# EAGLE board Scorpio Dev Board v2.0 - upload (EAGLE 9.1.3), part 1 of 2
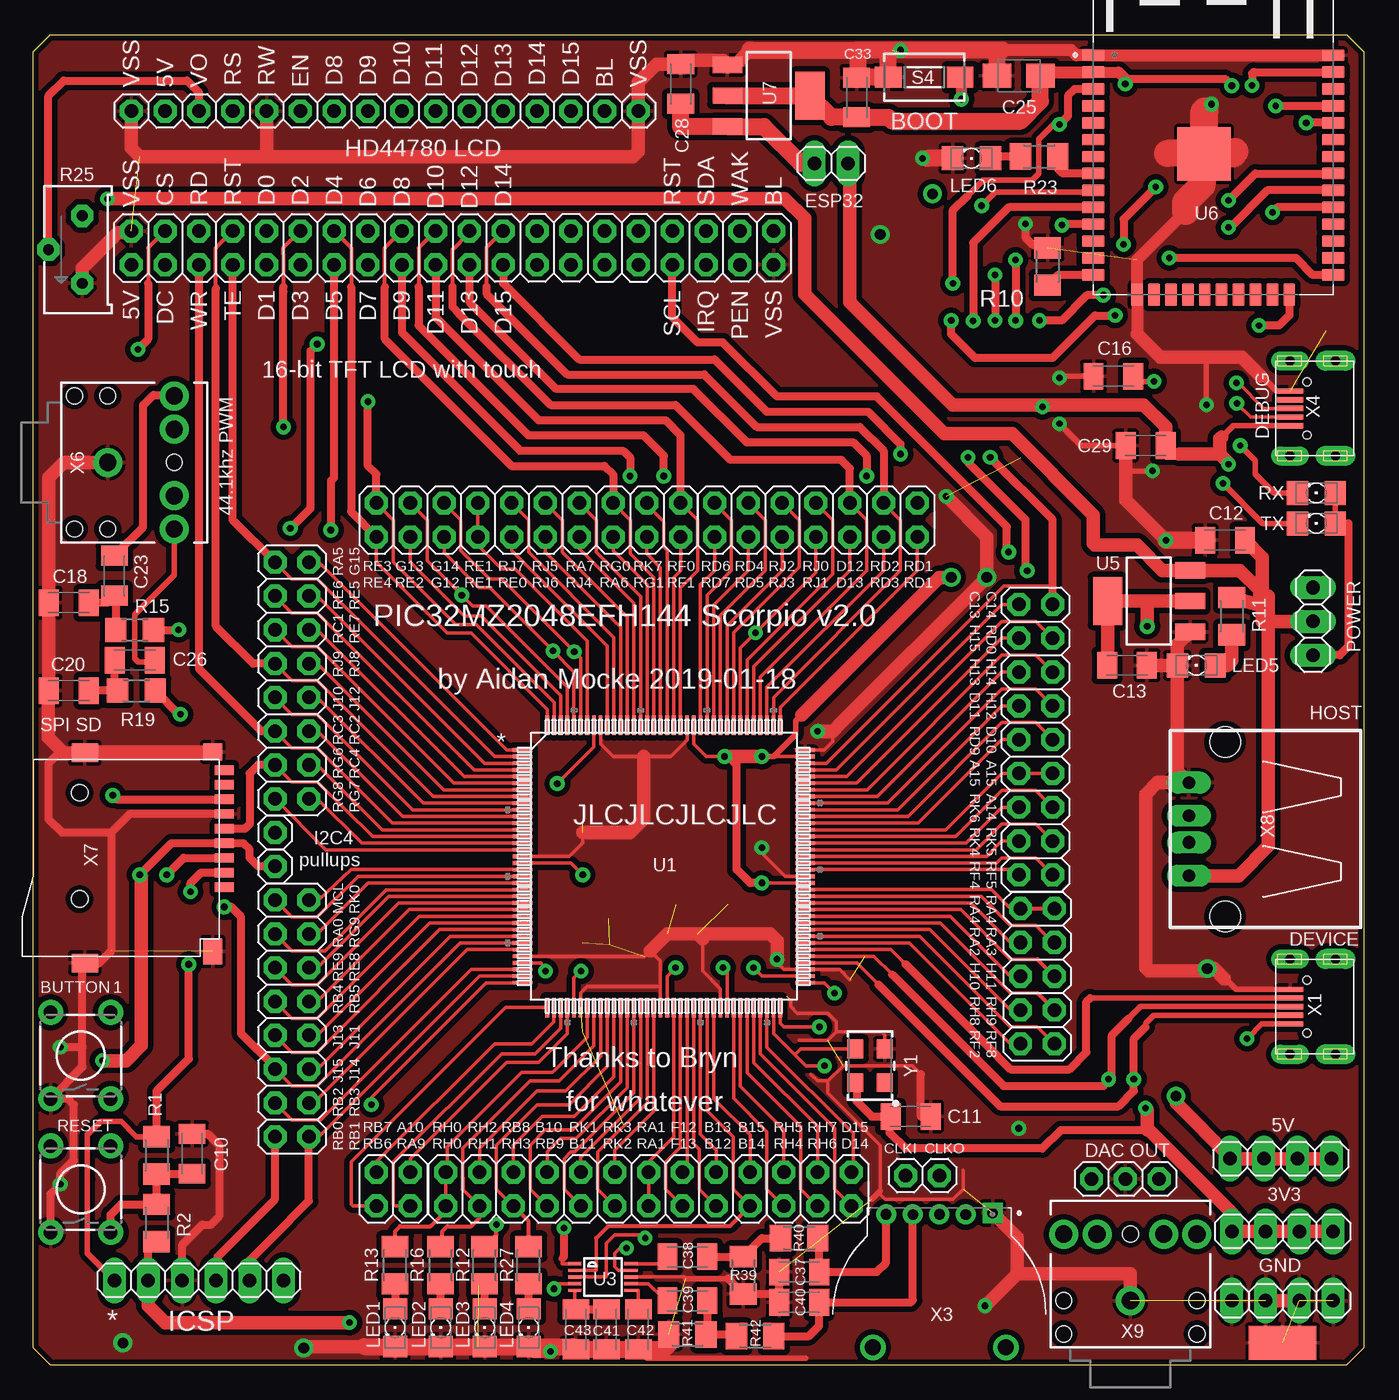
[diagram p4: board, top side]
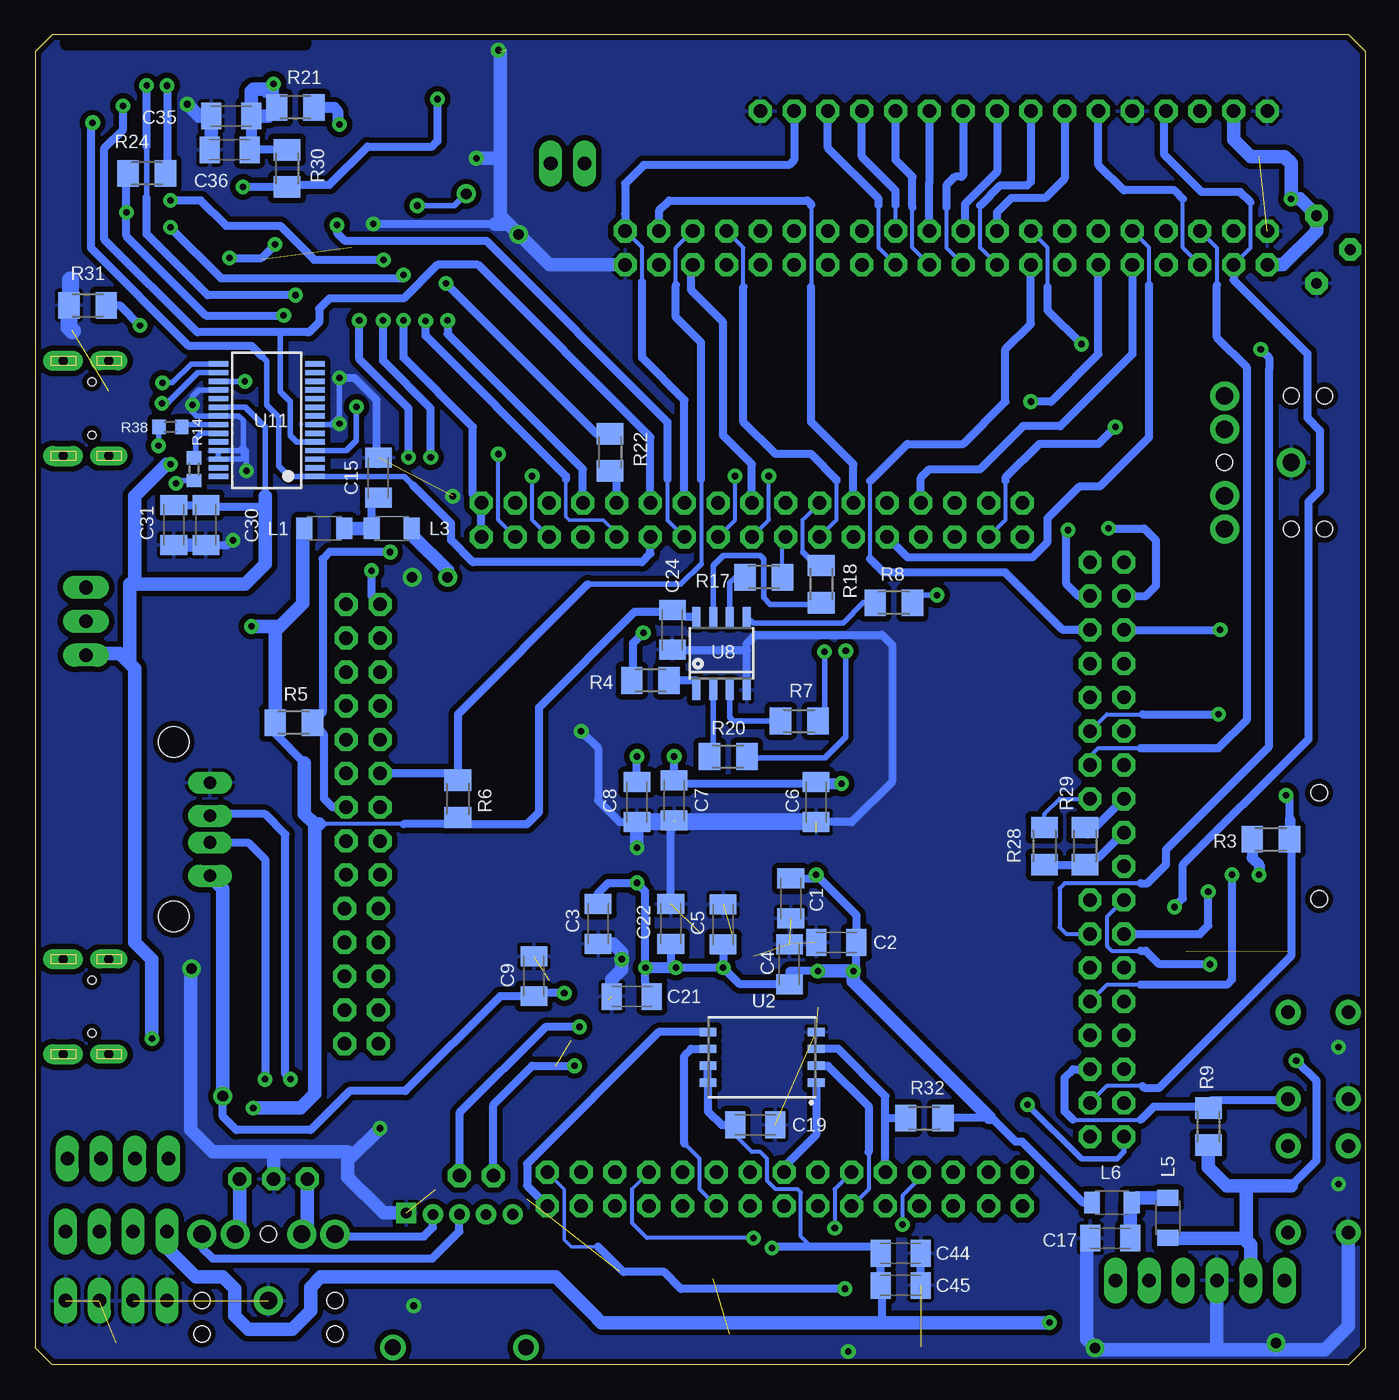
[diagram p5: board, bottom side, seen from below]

Size 99.95 x 99.95 mm. Coordinates in mm from the lower left corner, seen from the top.
Outline: 98.68,0 99.95,1.27 99.95,98.68 98.68,99.95 1.27,99.95 0,98.68 0,1.27 1.27,0 98.68,0
Copper layers (1*16): Top 0.035mm / dielectric 1.5mm / Bottom 0.035mm
Design rules "default *": minimum track width 10mil, minimum drill 19mil, track to track 7mil, track to pad 7mil, pad to pad 7mil, via to via 7mil, smd to smd 7mil, copper to edge 12mil, drill to drill 8mil, minimum pad ring 14mil, minimum via ring 12mil, stop-mask expansion 4mil, vias tented up to drill 0mil, thermal gap 10mil

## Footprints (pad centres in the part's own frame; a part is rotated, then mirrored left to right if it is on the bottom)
C1206K = smd 1.5 x 2: 1 -1.5,0; 2 1.5,0
B/3528-21W = smd 2.15 x 1.8: + 1.625,0; - -1.625,0
2X02 = drill 1.016 octagon: 1 -1.27,-1.27; 2 -1.27,1.27; 3 1.27,-1.27; 4 1.27,1.27
1X01 = drill 1.016 octagon: 1 0,0
2X07 = drill 1.016 octagon: 1 -7.62,-1.27; 2 -7.62,1.27; 3 -5.08,-1.27; 4 -5.08,1.27; 5 -2.54,-1.27; 6 -2.54,1.27; 7 0,-1.27; 8 0,1.27; 9 2.54,-1.27; 10 2.54,1.27; 11 5.08,-1.27; 12 5.08,1.27; 13 7.62,-1.27; 14 7.62,1.27
2X05 = drill 1.016 octagon: 1 -5.08,-1.27; 2 -5.08,1.27; 3 -2.54,-1.27; 4 -2.54,1.27; 5 0,-1.27; 6 0,1.27; 7 2.54,-1.27; 8 2.54,1.27; 9 5.08,-1.27; 10 5.08,1.27
2X20 = drill 1.016 octagon: 1 -24.13,-1.27; 2 -24.13,1.27; 3 -21.59,-1.27; 4 -21.59,1.27; 5 -19.05,-1.27; 6 -19.05,1.27; 7 -16.51,-1.27; 8 -16.51,1.27; 9 -13.97,-1.27; 10 -13.97,1.27; 11 -11.43,-1.27; 12 -11.43,1.27; 13 -8.89,-1.27; 14 -8.89,1.27; 15 -6.35,-1.27; 16 -6.35,1.27; 17 -3.81,-1.27; 18 -3.81,1.27; 19 -1.27,-1.27; 20 -1.27,1.27; 21 1.27,-1.27; 22 1.27,1.27; 23 3.81,-1.27; 24 3.81,1.27; 25 6.35,-1.27; 26 6.35,1.27; 27 8.89,-1.27; 28 8.89,1.27; 29 11.43,-1.27; 30 11.43,1.27; 31 13.97,-1.27; 32 13.97,1.27; 33 16.51,-1.27; 34 16.51,1.27; 35 19.05,-1.27; 36 19.05,1.27; 37 21.59,-1.27; 38 21.59,1.27; 39 24.13,-1.27; 40 24.13,1.27
2X08 = drill 1.016 octagon: 1 -8.89,-1.27; 2 -8.89,1.27; 3 -6.35,-1.27; 4 -6.35,1.27; 5 -3.81,-1.27; 6 -3.81,1.27; 7 -1.27,-1.27; 8 -1.27,1.27; 9 1.27,-1.27; 10 1.27,1.27; 11 3.81,-1.27; 12 3.81,1.27; 13 6.35,-1.27; 14 6.35,1.27; 15 8.89,-1.27; 16 8.89,1.27
2X03 = drill 1.016 octagon: 1 -2.54,-1.27; 2 -2.54,1.27; 3 0,-1.27; 4 0,1.27; 5 2.54,-1.27; 6 2.54,1.27
2X09 = drill 1.016 octagon: 1 -10.16,-1.27; 2 -10.16,1.27; 3 -7.62,-1.27; 4 -7.62,1.27; 5 -5.08,-1.27; 6 -5.08,1.27; 7 -2.54,-1.27; 8 -2.54,1.27; 9 0,-1.27; 10 0,1.27; 11 2.54,-1.27; 12 2.54,1.27; 13 5.08,-1.27; 14 5.08,1.27; 15 7.62,-1.27; 16 7.62,1.27; 17 10.16,-1.27; 18 10.16,1.27
2X10 = drill 1.016 octagon: 1 -11.43,-1.27; 2 -11.43,1.27; 3 -8.89,-1.27; 4 -8.89,1.27; 5 -6.35,-1.27; 6 -6.35,1.27; 7 -3.81,-1.27; 8 -3.81,1.27; 9 -1.27,-1.27; 10 -1.27,1.27; 11 1.27,-1.27; 12 1.27,1.27; 13 3.81,-1.27; 14 3.81,1.27; 15 6.35,-1.27; 16 6.35,1.27; 17 8.89,-1.27; 18 8.89,1.27; 19 11.43,-1.27; 20 11.43,1.27
1X04 = drill 1.016 long: 1 -3.81,0; 2 -1.27,0; 3 1.27,0; 4 3.81,0
1X03 = drill 1.016 long: 1 -2.54,0; 2 0,0; 3 2.54,0
1X16 = drill 1.016 octagon: 1 -19.05,0; 2 -16.51,0; 3 -13.97,0; 4 -11.43,0; 5 -8.89,0; 6 -6.35,0; 7 -3.81,0; 8 -1.27,0; 9 1.27,0; 10 3.81,0; 11 6.35,0; 12 8.89,0; 13 11.43,0; 14 13.97,0; 15 16.51,0; 16 19.05,0
1X06 = drill 1.016 long: 1 -6.35,0; 2 -3.81,0; 3 -1.27,0; 4 1.27,0; 5 3.81,0; 6 6.35,0
1X02 = drill 1.016 long: 1 -1.27,0; 2 1.27,0
L3216C = smd 1.2 x 1.6: 1 -1.5,0; 2 1.5,0
1206 = smd 1.6 x 1.803: A -1.422,0; C 1.422,0
SMD2,54-5,08 = smd 2.54 x 5.08: 1 0,0
M1206 = smd 1.6 x 2: 1 -1.4,0; 2 1.4,0
R0603 = smd 1 x 1.1: 1 -0.85,0; 2 0.85,0
R1206 = smd 1.6 x 1.803: 1 -1.422,0; 2 1.422,0
3386X = drill 0.813 pad 1.676 octagon: 1 2.54,0.635; 2 0,-1.905; 3 -2.54,0.635
TACTILE-PTH = drill 1.016 pad 1.88: 1 -3.251,2.261; 2 3.251,2.261; 3 -3.251,-2.261; 4 3.251,-2.261
DTSM-3 = smd 2 x 1.6: 1 -2.7,0; 2 2.7,0
LQFP144_20X20MC = smd 1.473 x 0.279: 1 -10.617,8.75; 2 -10.617,8.25; 3 -10.617,7.75; 4 -10.617,7.25; 5 -10.617,6.75; 6 -10.617,6.25; 7 -10.617,5.75; 8 -10.617,5.25; 9 -10.617,4.75; 10 -10.617,4.25; 11 -10.617,3.75; 12 -10.617,3.25; 13 -10.617,2.75; 14 -10.617,2.25; 15 -10.617,1.75; 16 -10.617,1.25; 17 -10.617,0.75; 18 -10.617,0.25; 19 -10.617,-0.25; 20 -10.617,-0.75; 21 -10.617,-1.25; 22 -10.617,-1.75; 23 -10.617,-2.25; 24 -10.617,-2.75; 25 -10.617,-3.25; 26 -10.617,-3.75; 27 -10.617,-4.25; 28 -10.617,-4.75; 29 -10.617,-5.25; 30 -10.617,-5.75; 31 -10.617,-6.25; 32 -10.617,-6.75; 33 -10.617,-7.25; 34 -10.617,-7.75; 35 -10.617,-8.25; 36 -10.617,-8.75; 73 10.617,-8.75; 74 10.617,-8.25; 75 10.617,-7.75; 76 10.617,-7.25; 77 10.617,-6.75; 78 10.617,-6.25; 79 10.617,-5.75; 80 10.617,-5.25; 81 10.617,-4.75; 82 10.617,-4.25; 83 10.617,-3.75; 84 10.617,-3.25; 85 10.617,-2.75; 86 10.617,-2.25; 87 10.617,-1.75; 88 10.617,-1.25; 89 10.617,-0.75; 90 10.617,-0.25; 91 10.617,0.25; 92 10.617,0.75; 93 10.617,1.25; 94 10.617,1.75; 95 10.617,2.25; 96 10.617,2.75; 97 10.617,3.25; 98 10.617,3.75; 99 10.617,4.25; 100 10.617,4.75; 101 10.617,5.25; 102 10.617,5.75; 103 10.617,6.25; 104 10.617,6.75; 105 10.617,7.25; 106 10.617,7.75; 107 10.617,8.25; 108 10.617,8.75 | smd 0.279 x 1.473: 37 -8.75,-10.617; 38 -8.25,-10.617; 39 -7.75,-10.617; 40 -7.25,-10.617; 41 -6.75,-10.617; 42 -6.25,-10.617; 43 -5.75,-10.617; 44 -5.25,-10.617; 45 -4.75,-10.617; 46 -4.25,-10.617; 47 -3.75,-10.617; 48 -3.25,-10.617; 49 -2.75,-10.617; 50 -2.25,-10.617; 51 -1.75,-10.617; 52 -1.25,-10.617; 53 -0.75,-10.617; 54 -0.25,-10.617; 55 0.25,-10.617; 56 0.75,-10.617; 57 1.25,-10.617; 58 1.75,-10.617; 59 2.25,-10.617; 60 2.75,-10.617; 61 3.25,-10.617; 62 3.75,-10.617; 63 4.25,-10.617; 64 4.75,-10.617; 65 5.25,-10.617; 66 5.75,-10.617; 67 6.25,-10.617; 68 6.75,-10.617; 69 7.25,-10.617; 70 7.75,-10.617; 71 8.25,-10.617; 72 8.75,-10.617; 109 8.75,10.617; 110 8.25,10.617; 111 7.75,10.617; 112 7.25,10.617; 113 6.75,10.617; 114 6.25,10.617; 115 5.75,10.617; 116 5.25,10.617; 117 4.75,10.617; 118 4.25,10.617; 119 3.75,10.617; 120 3.25,10.617; 121 2.75,10.617; 122 2.25,10.617; 123 1.75,10.617; 124 1.25,10.617; 125 0.75,10.617; 126 0.25,10.617; 127 -0.25,10.617; 128 -0.75,10.617; 129 -1.25,10.617; 130 -1.75,10.617; 131 -2.25,10.617; 132 -2.75,10.617; 133 -3.25,10.617; 134 -3.75,10.617; 135 -4.25,10.617; 136 -4.75,10.617; 137 -5.25,10.617; 138 -5.75,10.617; 139 -6.25,10.617; 140 -6.75,10.617; 141 -7.25,10.617; 142 -7.75,10.617; 143 -8.25,10.617; 144 -8.75,10.617
WSON8-Q2A = smd 0.635 x 1.27: 1 -1.905,-4.064; 2 -0.635,-4.064; 3 0.635,-4.064; 4 1.905,-4.064; 5 1.905,4.064; 6 0.635,4.064; 7 -0.635,4.064; 8 -1.905,4.064
MSOP10 = smd 0.25 x 1: 1 -1,-2.113; 2 -0.5,-2.113; 3 0,-2.113; 4 0.5,-2.113; 5 1,-2.113; 6 1,2.113; 7 0.5,2.113; 8 0,2.113; 9 -0.5,2.113; 10 -1,2.113
SOT223 = smd 1.219 x 2.235: 1 -2.311,-3.099; 2 0,-3.099; 3 2.311,-3.099 | smd 3.6 x 2.2: 4 0,3.099
MODULE_ESP-WROOM-32 = smd 1.7 x 0.9: 1 -9,8.255; 2 -9,6.985; 3 -9,5.715; 4 -9,4.445; 5 -9,3.175; 6 -9,1.905; 7 -9,0.635; 8 -9,-0.635; 9 -9,-1.905; 10 -9,-3.175; 11 -9,-4.445; 12 -9,-5.715; 13 -9,-6.985; 14 -9,-8.255; 25 9,-8.255; 26 9,-6.985; 27 9,-5.715; 28 9,-4.445; 29 9,-3.175; 30 9,-1.905; 31 9,-0.635; 32 9,0.635; 33 9,1.905; 34 9,3.175; 35 9,4.445; 36 9,5.715; 37 9,6.985; 38 9,8.255 | smd 4 x 4: 1.1 -0.7,0.845 | smd 0.9 x 1.7: 15 -5.715,-9.755; 16 -4.445,-9.755; 17 -3.175,-9.755; 18 -1.905,-9.755; 19 -0.635,-9.755; 20 0.635,-9.755; 21 1.905,-9.755; 22 3.175,-9.755; 23 4.445,-9.755; 24 5.715,-9.755
SOIC8 = smd 0.6 x 1.5: 1 -1.905,-2.75; 2 -0.635,-2.75; 3 0.635,-2.75; 4 1.905,-2.75; 5 1.905,2.75; 6 0.635,2.75; 7 -0.635,2.75; 8 -1.905,2.75
SSOP28 = smd 0.4 x 1.5: 1 -4.225,-3.625; 2 -3.575,-3.625; 3 -2.925,-3.625; 4 -2.275,-3.625; 5 -1.625,-3.625; 6 -0.975,-3.625; 7 -0.325,-3.625; 8 0.325,-3.625; 9 0.975,-3.625; 10 1.625,-3.625; 11 2.275,-3.625; 12 2.925,-3.625; 13 3.575,-3.625; 14 4.225,-3.625; 15 4.225,3.625; 16 3.575,3.625; 17 2.925,3.625; 18 2.275,3.625; 19 1.625,3.625; 20 0.975,3.625; 21 0.325,3.625; 22 -0.325,3.625; 23 -0.975,3.625; 24 -1.625,3.625; 25 -2.275,3.625; 26 -2.925,3.625; 27 -3.575,3.625; 28 -4.225,3.625
LCSC_MICRO_USB_4_LEGS = smd 1.95 x 0.4: D+ 3.225,0; D- 3.225,0.65; GND 3.225,-1.3; ID 3.225,-0.65; VBUS 3.225,1.3 | drill 0.7 pad 1.5 long: P$1 -0.177,3.575; P$2 -0.177,-3.575 | drill 0.7 pad 1.4 long: P$3 3.25,3.575; P$5 3.25,-3.575 | hole 0.6: 1.973,2; 1.973,-2
TRIM_A14061600UX0005 = drill 0.8 square: 1 -4,-7.6 | drill 0.8: 2 -1.988,-7.493; 3 0,-7.5; 4 1.992,-7.493; 5 4,-7.5 | drill 1.2: NC1 -5,2.5; NC2 5,2.5
AUDIO-JACK = drill 1.3 pad 2.184: RING 5,5; RSH 5,2.5; SLEEVE 0,0; TIP 5,-5; TSH 5,-2.5 | hole 1.2: 0,5; -2.5,5; -2.5,-5; 0,-5; 5,0
SD-MMC_TF-PULL = smd 0.7 x 1.4: 1 -2.2,-7.62; 2 -1.1,-7.62; 3 0,-7.62; 4 1.1,-7.62; 5 2.2,-7.62; 6 3.3,-7.62; 7 4.4,-7.62; 8 5.5,-7.62; 9 6.6,-7.62 | smd 1.4 x 2: S1 -7.9,2.85; S2 7.9,2.85 | smd 1.28 x 1.4: S3 7.96,-6.75 | smd 1.95 x 1.4: S4 -7.025,-6.75 | hole 1.25: -3.1,3.25; 4.9,3.25
PN87520 = drill 0.95 long: 1 -3.5,2.71; 2 -1,2.71; 3 1,2.71; 4 3.5,2.71 | hole 2.3: -6.57,0; 6.57,0
OSCILLATOR-SMD-5X3.2 = smd 1.397 x 1.194: 1 -1.27,-1.1; 2 1.27,-1.1; 3 1.27,1.1; 4 -1.27,1.1

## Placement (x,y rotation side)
C1  0.1uF  [C1206K]  43.18,35.05 270 bottom
C2  0.1uF  [C1206K]  39.75,31.75 180 bottom
C3  0.1uF  [C1206K]  57.66,33.15 270 bottom
C4  0.1uF  [C1206K]  43.28,30.1 90 bottom
C5  0.1uF  [C1206K]  48.26,33.1 90 bottom
C6  0.1uF  [C1206K]  41.27,42.29 270 bottom
C7  0.1uF  [C1206K]  51.94,42.42 270 bottom
C8  0.1uF  [C1206K]  54.74,42.29 270 bottom
C9  0.1uF  [C1206K]  62.48,29.21 90 bottom
C10  0.1uF  [C1206K]  11.94,15.88 90 top
C11  0.01uF  [C1206K]  65.91,18.67 0 top
C12  10uF  [C1206K]  89.53,61.98 180 top
C13  10uF  [C1206K]  82.17,52.58 0 top
C15  0.01uF  [C1206K]  74.17,66.67 90 bottom
C16  0.1uF  [C1206K]  81.15,74.3 180 top
C17  0.01uF  [C1206K]  19.18,9.53 180 bottom
C18  0.1uF  [C1206K]  2.67,57.28 0 top
C19  0.1uF  [C1206K]  45.85,18.03 0 bottom
C20  0.1uF  [C1206K]  2.67,50.67 0 top
C21  0.1uF  [C1206K]  55.12,27.69 180 bottom
C22  0.1uF  [C1206K]  52.2,33.15 90 bottom
C23  0.1uF  [C1206K]  6.1,59.31 90 top
C24  0.1uF  [C1206K]  52.07,55.25 270 bottom
C25  100uF  [B/3528-21W]  74.04,96.9 0 top
C26  0.1uF  [C1206K]  7.62,52.96 0 top
C28  10uF  [C1206K]  48.64,96.27 90 top
C29  0.1uF  [C1206K]  83.57,69.09 180 top
C30  10nF  [C1206K]  87.12,63.12 270 bottom
C31  10uF  [C1206K]  89.53,63.12 270 bottom
C33  10uF  [C1206K]  61.85,95.25 90 top
C35  10uF  [C1206K]  85.22,93.85 180 bottom
C36  0.1uF  [C1206K]  85.34,91.31 180 bottom
C37  0.22uF  [C1206K]  57.53,6.98 180 top
C38  3.3uF  [C1206K]  49.15,8.13 0 top
C39  3.3uF  [C1206K]  49.15,4.83 0 top
C40  0.22uF  [C1206K]  57.53,4.7 180 top
C41  0.1uF  [C1206K]  43.05,2.67 270 top
C42  10uF  [C1206K]  45.47,2.67 270 top
C43  10uF  [C1206K]  40.77,2.67 270 top
C44  0.1uF  [C1206K]  34.92,8.38 0 bottom
C45  10uF  [C1206K]  34.92,5.97 0 bottom
JP1  [2X02]  27.05,13.21 180 top
JP2  [1X01]  68.07,14.22 0 top
JP3  [2X07]  58.8,63.5 0 top
JP4  [2X05]  75.44,29.21 90 top
JP5  [2X20]  31.5,83.95 0 top
JP6  [2X08]  19.43,51.44 270 top
JP7  [2X03]  58.93,13.21 180 top
JP8  [2X09]  75.31,46.99 90 top
JP9  [2X10]  37.21,63.5 0 top
JP10  [1X01]  65.53,14.22 0 top
JP11  [1X01]  82.04,13.97 0 top
JP12  [1X04]  93.73,15.49 0 top
JP13  [1X01]  18.16,40 0 top
JP14  [1X03]  96.14,55.88 270 top
JP15  [2X08]  19.43,26.04 270 top
JP16  [1X04]  93.85,10.03 0 top
JP17  [1X04]  93.85,4.83 0 top
JP18  [1X01]  18.16,37.47 0 top
JP19  [2X10]  42.42,13.21 180 top
JP20  1X16  [1X16]  26.42,94.23 0 top
JP22  [1X06]  12.45,6.35 180 top
JP23  [1X01]  84.58,13.97 0 top
JP24  [1X02]  59.94,90.3 0 top
JP25  [1X01]  79.5,13.97 0 top
L1  L4  [L3216C]  78.23,62.87 0 bottom
L3  L3  [L3216C]  73.15,62.87 180 bottom
L5  [L3216C]  14.86,11.05 90 bottom
L6  [L3216C]  19.05,12.19 0 bottom
LED1  [1206]  27.18,2.79 270 top
LED2  [1206]  30.61,2.79 270 top
LED3  [1206]  33.91,2.79 270 top
LED4  [1206]  37.21,2.79 270 top
LED5  .PWR  [1206]  87.38,52.58 180 top
LED6  [1206]  70.48,90.68 180 top
PAD4  [SMD2,54-5,08]  93.85,1.65 90 top
R1  1k  [M1206]  9.27,15.75 90 top
R2  10k  [M1206]  9.27,10.67 90 top
R3  10k  [M1206]  7.11,39.5 180 bottom
R4  50  [M1206]  53.72,51.44 0 bottom
R5  10k  [M1206]  80.52,48.26 0 bottom
R6  10k  [M1206]  68.2,42.55 90 bottom
R7  50  [M1206]  42.54,48.39 180 bottom
R8  50  [M1206]  35.43,57.28 0 bottom
R9  10k  [M1206]  11.81,17.91 90 bottom
R10  10k  [M1206]  76.2,82.55 90 top
R11  1k  [M1206]  90.04,56.26 90 top
R12  1k  [M1206]  33.91,7.49 270 top
R13  1k  [M1206]  27.18,7.49 270 top
R14  330  [R0603]  88.01,67.31 270 bottom
R15  75  [R1206]  7.62,55.25 180 top
R16  1k  [M1206]  30.61,7.49 270 top
R17  50  [M1206]  45.21,59.18 0 bottom
R18  50  [M1206]  40.89,58.67 90 bottom
R19  39  [R1206]  7.75,50.67 180 top
R20  50  [M1206]  47.88,45.72 180 bottom
R21  10k  [M1206]  80.39,94.49 0 bottom
R22  10k  [M1206]  56.77,68.58 90 bottom
R23  1K  [M1206]  75.56,90.81 180 top
R24  10k  [M1206]  91.57,89.54 0 bottom
R25  [3386X]  3.05,83.82 270 top
R27  1k  [M1206]  37.21,7.49 270 top
R28  10k  [M1206]  24.13,38.99 90 bottom
R29  10k  [M1206]  21.08,38.99 90 bottom
R30  10k  [M1206]  81.03,89.92 90 bottom
R31  10k  [M1206]  96.01,79.63 180 bottom
R32  10k  [M1206]  33.15,18.54 180 bottom
R38  330  [R0603]  89.79,70.48 180 bottom
R39  10k  [M1206]  53.34,6.73 90 top
R40  470  [M1206]  57.53,9.53 180 top
R41  10k  [M1206]  49.15,2.29 180 top
R42  470  [M1206]  54.23,2.16 180 top
RX  [1206]  96.39,65.53 180 top
S1  SWITCH-MOMENTARY-2PTH  [TACTILE-PTH]  3.56,13.21 90 top
S2  SWITCH-MOMENTARY-2PTH  [TACTILE-PTH]  3.56,23.24 90 top
S4  DTSM-3  [DTSM-3]  66.93,96.77 0 top
TX  [1206]  96.39,63.25 180 top
U1  PIC32MZXXXXEC(G/H/M)144-I/PL  [LQFP144_20X20MC]  47.37,37.47 0 top
U2  SST25VF064C-Q2  [WSON8-Q2A]  45.34,23.11 90 bottom
U3  [MSOP10]  42.8,6.6 270 top
U5  [SOT223]  83.82,57.4 90 top
U6  ESP-WROOM-32  [MODULE_ESP-WROOM-32]  88.65,90.17 0 top
U7  [SOT223]  55.24,95.38 270 top
U8  VTI7064  [SOIC8]  48.39,53.47 0 bottom
U11  FT232RL  [SSOP28]  82.55,70.99 90 bottom
X1  USB4LEGS  [LCSC_MICRO_USB_4_LEGS]  97.66,26.92 180 top
X3  THUMBPOT  [TRIM_A14061600UX0005]  68.07,3.81 180 top
X4  LCSC_MICRO_USB_4_LEGS  [LCSC_MICRO_USB_4_LEGS]  97.66,71.88 180 top
X6  AUDIO_JACK_3.5MM_PTH  [AUDIO-JACK]  5.59,67.82 0 top
X7  SD-MMC_TF-HOLDER  [SD-MMC_TF-PULL]  6.73,38.1 90 top
X8  [PN87520]  89.53,40.26 90 top
X9  AUDIO_JACK_3.5MM_PTH  [AUDIO-JACK]  82.42,4.83 90 top
Y1  OSCILLATORSMD-5X3  [OSCILLATOR-SMD-5X3.2]  62.87,22.48 90 top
